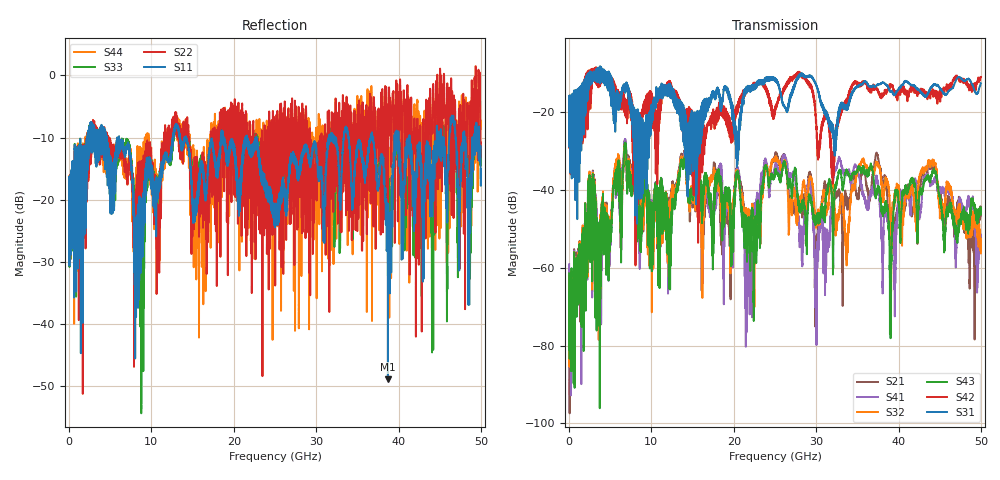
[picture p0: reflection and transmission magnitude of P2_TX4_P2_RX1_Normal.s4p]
!Keysight Technologies,N5225B,MY57041031,A.13.20.10
!Date: Friday, May 31, 2019 11:27:37
!Correction: S11(Full 4 Port(1,2,3,4))
!S12(Full 4 Port(1,2,3,4))
!S13(Full 4 Port(1,2,3,4))
!S14(Full 4 Port(1,2,3,4))
!S21(Full 4 Port(1,2,3,4))
!S22(Full 4 Port(1,2,3,4))
!S23(Full 4 Port(1,2,3,4))
!S24(Full 4 Port(1,2,3,4))
!S31(Full 4 Port(1,2,3,4))
!S32(Full 4 Port(1,2,3,4))
!S33(Full 4 Port(1,2,3,4))
!S34(Full 4 Port(1,2,3,4))
!S41(Full 4 Port(1,2,3,4))
!S42(Full 4 Port(1,2,3,4))
!S43(Full 4 Port(1,2,3,4))
!S44(Full 4 Port(1,2,3,4))
!S4P File: Measurements: <S11,S12,S13,S14>,
!<S21,S22,S23,S24>,
!<S31,S32,S33,S34>,
!<S41,S42,S43,S44>:
# Hz S  dB  R 50.0
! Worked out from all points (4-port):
!   5000 points, 10 MHz to 50 GHz, reference 50 ohm
!   strongest paths, dB at 10 MHz, 12.51 GHz, 25.01 GHz, 37.51 GHz, 50 GHz:
!     S31: -19.3, -14.3, -11.3, -12.8, -12.5
!     S42: -19.4, -14.3, -20.1, -14.6, -10.9
!     S43: -61.4, -44.7, -35.6, -39.2, -44.5
!     S32: -62.1, -40.9, -32.1, -33.7, -56.3
!     S41: -59.0, -44.2, -33.6, -38.1, -53.1
!     S21: -61.4, -40.2, -31.1, -31.6, -46.5
!   lowest |S11| = -48.9 dB at 38.71 GHz (marker M1), VSWR 1.01, Z = 49.6 - j0.0629 ohm
!   |S11| at or under -10 dB: 6.073 GHz to 12.61 GHz (6.542 GHz wide, 70 % of centre); 14.21 GHz to 18.43 GHz (4.227 GHz wide, 25.9 % of centre); 22.71 GHz to 31.52 GHz (8.806 GHz wide, 32.5 % of centre)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
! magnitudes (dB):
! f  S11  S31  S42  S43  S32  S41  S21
! 10 MHz  -18.9  -19.3  -19.4  -61.4  -62.1  -59.0  -61.4
! 6.75 GHz  -12.5  -14.5  -19.7  -28.9  -29.2  -27.8  -28.3
! 20.44 GHz  -17.9  -28.8  -19.8  -35.4  -35.3  -34.4  -34.7
! 22.1 GHz  -13.0  -13.2  -13.5  -52.4  -47.5  -50.3  -61.0
! 25.11 GHz  -23.1  -11.4  -18.8  -34.9  -31.3  -32.7  -30.2
! 38.71 GHz  -48.9  -13.5  -14.0  -44.8  -38.2  -46.7  -44.1
! 50 GHz  -15.1  -12.5  -10.9  -44.5  -56.3  -53.1  -46.5
